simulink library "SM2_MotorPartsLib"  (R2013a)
settings: Solver=ode45  StartTime=0.0  StopTime=10.0  RelTol=1e-3
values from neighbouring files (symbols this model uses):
  m = v*BEAM.rho    [FlexBeamModelConstruct2.m]    (also in FlexBeamModelConstruct3.m = BEAM.rho*v; FlexBeam_1D_Construct.m = REF.m/REF.l*a.*(linspace(1-OPT.MassBiais+1e-6,1+OPT.MassBiai; FlexBeam_3D_Construct.m = REF.m/REF.l*a.*(linspace(1-OPT.MassBiais+1e-6,1+OPT.MassBiai; FreeFlexBeam_3D_Construct.m = REF.m/REF.l*a.*tmp2)
  N = D(1)+(H4^2+H3^2)/H2^2-(E(1)*H4+F(1)*H3)/H2    [MGD.m]    (also in MGD2.m)
  s = -sign(imag(KGZ_fr_tmp))    [LinprogReguliOptimFunc_1.m]    (also in LinprogReguliOptimFunc_2.m; LinprogReguliOptimFunc_1 - Copie.m)
  X = cos(phi(i))*x+sin(phi(i))*y    [MGI.m]
  Y = fft(y(:,i),NFFT)/L    [fft_bis.m]    (also in MGI.m = -sin(phi(i))*x+cos(phi(i))*y)
  Z = z    [MGI.m]
undefined symbols (not defined in the file or in its folder): AxisID, deg, kg, rad, SimParam
libraries: sm_lib x46, nesl_utility x13

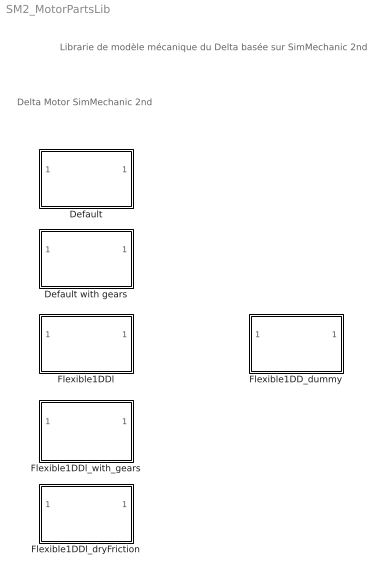
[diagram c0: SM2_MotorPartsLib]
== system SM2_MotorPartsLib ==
  note: Delta Motor SimMechanic 2nd
  note: Librarie de modèle mécanique du Delta basée sur SimMechanic 2nd
  Default : Subsystem  InitFcn=SimParam.Motor=RigidMotor_paramInitFnc(RawParam,IC);  VariantControl=motorVarDefault
  Default with gears : Subsystem  InitFcn=SimParam.Motor=RigidMotor_paramInitFnc(RawParam,IC);  VariantControl=motorVarGear
  Flexible1DD_dummy : Subsystem  InitFcn=SimParam.Motor=flexMotor_paramInitFnc(RawParam,IC);  VariantControl=motorVarFlex1
  Flexible1DDl : Subsystem  InitFcn=SimParam.Motor=flexMotor_paramInitFnc(RawParam,IC);  VariantControl=motorVarFlex1
  Flexible1DDl_dryFriction : Subsystem  InitFcn=SimParam.Motor=flexMotor_paramInitFnc(RawParam,IC);  VariantControl=motorVarFlex1
  Flexible1DDl_with_gears : Subsystem  InitFcn=SimParam.Motor=flexMotor_paramInitFnc(RawParam,IC);  VariantControl=motorVarFlex1

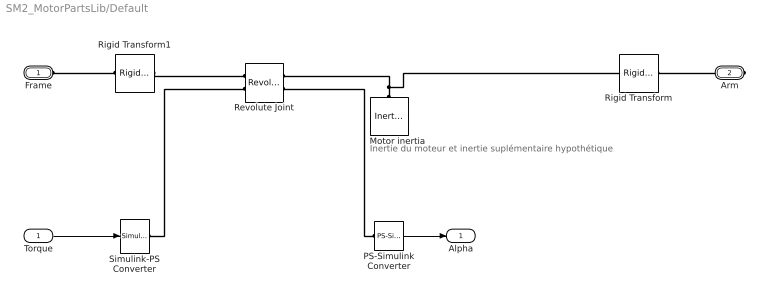
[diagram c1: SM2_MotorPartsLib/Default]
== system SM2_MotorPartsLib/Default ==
  note: Inertie du moteur et inertie suplémentaire hypothétique
  Torque : Inport
  Motor inertia : sm_lib/Body Elements/Inertia  InertiaType=Custom  Mass=1  MassUnits=kg  CenterOfMass=[0 0 0]  CenterOfMassUnits=m  MomentsOfInertia=(SimParam.Motor.I+SimParam.Motor.ISup).*[1 1 1]  MomentsOfInertiaUnits=kg*m^2  ProductsOfInertia=[0 0 0]  ProductsOfInertiaUnits=kg*m^2  BlockFunction=simmechanics.library.body_elements.inertia
  PS-Simulink Converter : nesl_utility/PS-Simulink Converter  PhysicalDomain=network_engine_domain  SubClassName=ps_output  LeftPortType=input  RightPortType=output  PseudoPeriodic=off  Frequencies=[]  Unit=1  AffineConversion=off
  Revolute Joint : sm_lib/Joints/Revolute Joint  SenseConstraintForceX=off  SenseConstraintForceY=off  SenseConstraintForceZ=off  SenseConstraintTorqueX=off  SenseConstraintTorqueY=off  SenseConstraintTorqueZ=off  ConstraintWrenchDir=FollowerOnBase  ConstraintWrenchFrame=BaseFrame  EquilibriumPosition=SimParam.Motor.Alpha(AxisID)  EquilibriumPositionUnits=rad  SpringStiffness=SimParam.Motor.kSup  SpringStiffnessUnits=N*m/rad  DampingCoefficient=SimParam.Motor.c  DampingCoefficientUnits=N*m/(rad/s)  ActuationMode=TorqueForceActuation  SensePosition=on  SenseVelocity=off  SenseAcceleration=off  SenseTorqueForce=off  PositionTargetValue=SimParam.Motor.Alpha(AxisID)  PositionTargetValueUnits=rad  PositionTargetSpecify=on  PositionTargetPriority=High  VelocityTargetValue=0  VelocityTargetValueUnits=rad/s  VelocityTargetSpecify=on  VelocityTargetPriority=High  BlockFunction=simmechanics.library.joints.revolute_joint
  Rigid Transform : sm_lib/Frames and  Transforms/Rigid  Transform  TranslationMethod=None  TranslationLengthUnit=m  TranslationStandardAxis=+Z  TranslationStandardOffset=0  TranslationCartesianOffset=[0 0 0]  TranslationROffset=0.2  TranslationROffsetUnits=m  TranslationZOffset=0  TranslationZOffsetUnits=m  TranslationThetaOffset=0  TranslationThetaOffsetUnits=deg  RotationMethod=AlignedAxes  RotationAngleUnits=rad  RotationStandardAxis=+Y  RotationAngle=0.2  RotationArbitraryAxis=[0 0 1]  FollAlignAxisA=+Y  BaseAlignAxisA=+Z  FollAlignAxisB=+X  BaseAlignAxisB=+X  BlockFunction=simmechanics.library.frames_transforms.rigid_transform
  Rigid Transform1 : sm_lib/Frames and  Transforms/Rigid  Transform  TranslationMethod=None  TranslationLengthUnit=m  TranslationStandardAxis=+Z  TranslationStandardOffset=0  TranslationCartesianOffset=[0 0 0]  TranslationROffset=0.2  TranslationROffsetUnits=m  TranslationZOffset=0  TranslationZOffsetUnits=m  TranslationThetaOffset=0  TranslationThetaOffsetUnits=deg  RotationMethod=AlignedAxes  RotationAngleUnits=rad  RotationStandardAxis=+Y  RotationAngle=0.2  RotationArbitraryAxis=[0 0 1]  FollAlignAxisA=+Z  BaseAlignAxisA=+Y  FollAlignAxisB=+X  BaseAlignAxisB=+X  BlockFunction=simmechanics.library.frames_transforms.rigid_transform
  Simulink-PS Converter : nesl_utility/Simulink-PS Converter  PhysicalDomain=network_engine_domain  SubClassName=ps_input  LeftPortType=input  RightPortType=output  PseudoPeriodic=off  Frequencies=[]  NoiseDistribution=none  NoiseParameters=[]  Unit=1  AffineConversion=off  InputFiltering=off  SimscapeFilterOrder=1  InputFilterTimeConstant=0.001  UdotUserProvided=1
  Frame : PMIOPort  Port=1  Side=Left
  Arm : PMIOPort  Port=2  Side=Right
  Alpha : Outport
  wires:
  PS-Simulink Converter/1 -> Alpha/1
  Torque/1 -> Simulink-PS Converter/1
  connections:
  Simulink-PS Converter/RConn1 -- Revolute Joint/LConn2
  Rigid Transform1/RConn1 -- Revolute Joint/LConn1
  Motor inertia/RConn1 -- Revolute Joint/RConn1 -- Rigid Transform/LConn1
  PS-Simulink Converter/LConn1 -- Revolute Joint/RConn2
  Rigid Transform1/LConn1 -- Frame/RConn1
  Arm/RConn1 -- Rigid Transform/RConn1

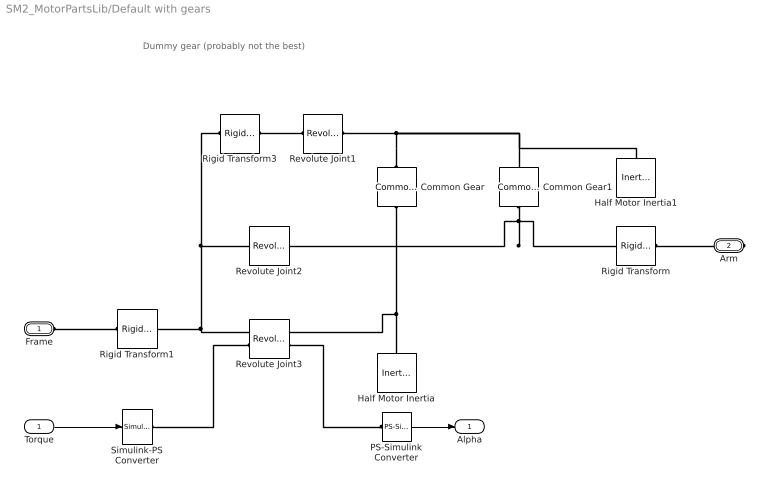
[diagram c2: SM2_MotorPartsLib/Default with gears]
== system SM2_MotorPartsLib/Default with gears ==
  note: Dummy gear (probably not the best)
  Torque : Inport
  Common Gear : sm_lib/Gears, Couplings and Drives/Gears/Common Gear  GearType=External  SpecificationType=CenterDistanceRatio  CenterDistance=0.01  CenterDistanceUnits=m  GearRatio=1  BaseGearRadius=10  BaseGearRadiusUnits=cm  FollGearRadius=10  FollGearRadiusUnits=cm  AssemblyGearRotation=Free  BlockFunction=simmechanics.library.gears_couplings_drives.gears.common_gear
  Common Gear1 : sm_lib/Gears, Couplings and Drives/Gears/Common Gear  GearType=External  SpecificationType=CenterDistanceRatio  CenterDistance=0.01  CenterDistanceUnits=m  GearRatio=SimParam.Motor.i  BaseGearRadius=10  BaseGearRadiusUnits=cm  FollGearRadius=10  FollGearRadiusUnits=cm  AssemblyGearRotation=Free  BlockFunction=simmechanics.library.gears_couplings_drives.gears.common_gear
  Half Motor Inertia : sm_lib/Body Elements/Inertia  InertiaType=Custom  Mass=1  MassUnits=kg  CenterOfMass=[0 0 0]  CenterOfMassUnits=m  MomentsOfInertia=0.5.*SimParam.Motor.I.*[1 1 1]  MomentsOfInertiaUnits=kg*m^2  ProductsOfInertia=[0 0 0]  ProductsOfInertiaUnits=kg*m^2  BlockFunction=simmechanics.library.body_elements.inertia
  Half Motor Inertia1 : sm_lib/Body Elements/Inertia  InertiaType=Custom  Mass=1  MassUnits=kg  CenterOfMass=[0 0 0]  CenterOfMassUnits=m  MomentsOfInertia=0.5.*SimParam.Motor.I.*[1 1 1]  MomentsOfInertiaUnits=kg*m^2  ProductsOfInertia=[0 0 0]  ProductsOfInertiaUnits=kg*m^2  BlockFunction=simmechanics.library.body_elements.inertia
  PS-Simulink Converter : nesl_utility/PS-Simulink Converter  PhysicalDomain=network_engine_domain  SubClassName=ps_output  LeftPortType=input  RightPortType=output  PseudoPeriodic=off  Frequencies=[]  Unit=1  AffineConversion=off
  Revolute Joint1 : sm_lib/Joints/Revolute Joint  SenseConstraintForceX=off  SenseConstraintForceY=off  SenseConstraintForceZ=off  SenseConstraintTorqueX=off  SenseConstraintTorqueY=off  SenseConstraintTorqueZ=off  ConstraintWrenchDir=FollowerOnBase  ConstraintWrenchFrame=BaseFrame  EquilibriumPosition=0  EquilibriumPositionUnits=rad  SpringStiffness=0  SpringStiffnessUnits=N*m/rad  DampingCoefficient=0  DampingCoefficientUnits=N*m/(rad/s)  ActuationMode=NoActuation  SensePosition=off  SenseVelocity=off  SenseAcceleration=off  SenseTorqueForce=off  PositionTargetValue=SimParam.Motor.Alpha(AxisID)  PositionTargetValueUnits=rad  PositionTargetSpecify=on  PositionTargetPriority=High  VelocityTargetValue=0  VelocityTargetValueUnits=deg/s  VelocityTargetSpecify=off  VelocityTargetPriority=High  BlockFunction=simmechanics.library.joints.revolute_joint
  Revolute Joint2 : sm_lib/Joints/Revolute Joint  SenseConstraintForceX=off  SenseConstraintForceY=off  SenseConstraintForceZ=off  SenseConstraintTorqueX=off  SenseConstraintTorqueY=off  SenseConstraintTorqueZ=off  ConstraintWrenchDir=FollowerOnBase  ConstraintWrenchFrame=BaseFrame  EquilibriumPosition=0  EquilibriumPositionUnits=rad  SpringStiffness=0  SpringStiffnessUnits=N*m/rad  DampingCoefficient=0  DampingCoefficientUnits=N*m/(rad/s)  ActuationMode=NoActuation  SensePosition=off  SenseVelocity=off  SenseAcceleration=off  SenseTorqueForce=off  PositionTargetValue=SimParam.Motor.Alpha(AxisID)  PositionTargetValueUnits=rad  PositionTargetSpecify=on  PositionTargetPriority=High  VelocityTargetValue=0  VelocityTargetValueUnits=deg/s  VelocityTargetSpecify=off  VelocityTargetPriority=High  BlockFunction=simmechanics.library.joints.revolute_joint
  Revolute Joint3 : sm_lib/Joints/Revolute Joint  SenseConstraintForceX=off  SenseConstraintForceY=off  SenseConstraintForceZ=off  SenseConstraintTorqueX=off  SenseConstraintTorqueY=off  SenseConstraintTorqueZ=off  ConstraintWrenchDir=FollowerOnBase  ConstraintWrenchFrame=BaseFrame  EquilibriumPosition=SimParam.IC.Alpha(AxisID)  EquilibriumPositionUnits=rad  SpringStiffness=SimParam.Motor.kSup  SpringStiffnessUnits=N*m/rad  DampingCoefficient=SimParam.Motor.c  DampingCoefficientUnits=N*m/(rad/s)  ActuationMode=TorqueForceActuation  SensePosition=on  SenseVelocity=off  SenseAcceleration=off  SenseTorqueForce=off  PositionTargetValue=SimParam.Motor.Alpha(AxisID)  PositionTargetValueUnits=rad  PositionTargetSpecify=on  PositionTargetPriority=High  VelocityTargetValue=0  VelocityTargetValueUnits=deg/s  VelocityTargetSpecify=off  VelocityTargetPriority=High  BlockFunction=simmechanics.library.joints.revolute_joint
  Rigid Transform : sm_lib/Frames and  Transforms/Rigid  Transform  TranslationMethod=None  TranslationLengthUnit=m  TranslationStandardAxis=+Z  TranslationStandardOffset=0  TranslationCartesianOffset=[0 0 0]  TranslationROffset=0.2  TranslationROffsetUnits=m  TranslationZOffset=0  TranslationZOffsetUnits=m  TranslationThetaOffset=0  TranslationThetaOffsetUnits=deg  RotationMethod=AlignedAxes  RotationAngleUnits=rad  RotationStandardAxis=+Y  RotationAngle=0.2  RotationArbitraryAxis=[0 0 1]  FollAlignAxisA=+Y  BaseAlignAxisA=+Z  FollAlignAxisB=+X  BaseAlignAxisB=+X  BlockFunction=simmechanics.library.frames_transforms.rigid_transform
  Rigid Transform1 : sm_lib/Frames and  Transforms/Rigid  Transform  TranslationMethod=None  TranslationLengthUnit=m  TranslationStandardAxis=+Z  TranslationStandardOffset=0  TranslationCartesianOffset=[0 0 0]  TranslationROffset=0.2  TranslationROffsetUnits=m  TranslationZOffset=0  TranslationZOffsetUnits=m  TranslationThetaOffset=0  TranslationThetaOffsetUnits=deg  RotationMethod=AlignedAxes  RotationAngleUnits=rad  RotationStandardAxis=+Y  RotationAngle=0.2  RotationArbitraryAxis=[0 0 1]  FollAlignAxisA=+Z  BaseAlignAxisA=+Y  FollAlignAxisB=+X  BaseAlignAxisB=+X  BlockFunction=simmechanics.library.frames_transforms.rigid_transform
  Rigid Transform3 : sm_lib/Frames and  Transforms/Rigid  Transform  TranslationMethod=Cartesian  TranslationLengthUnit=m  TranslationStandardAxis=+Z  TranslationStandardOffset=0  TranslationCartesianOffset=[0 .01 0]  TranslationROffset=0.2  TranslationROffsetUnits=m  TranslationZOffset=0  TranslationZOffsetUnits=m  TranslationThetaOffset=0  TranslationThetaOffsetUnits=deg  RotationMethod=None  RotationAngleUnits=rad  RotationStandardAxis=+Z  RotationAngle=SimParam.IC.Alpha(AxisID)  RotationArbitraryAxis=[0 0 1]  FollAlignAxisA=+Z  BaseAlignAxisA=+Y  FollAlignAxisB=+X  BaseAlignAxisB=+X  BlockFunction=simmechanics.library.frames_transforms.rigid_transform
  Simulink-PS Converter : nesl_utility/Simulink-PS Converter  PhysicalDomain=network_engine_domain  SubClassName=ps_input  LeftPortType=input  RightPortType=output  PseudoPeriodic=off  Frequencies=[]  NoiseDistribution=none  NoiseParameters=[]  Unit=1  AffineConversion=off  InputFiltering=off  SimscapeFilterOrder=1  InputFilterTimeConstant=0.001  UdotUserProvided=1
  Frame : PMIOPort  Port=1  Side=Left
  Arm : PMIOPort  Port=2  Side=Right
  Alpha : Outport
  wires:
  PS-Simulink Converter/1 -> Alpha/1
  Torque/1 -> Simulink-PS Converter/1
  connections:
  Revolute Joint3/LConn2 -- Simulink-PS Converter/RConn1
  Rigid Transform3/LConn1 -- Revolute Joint3/LConn1 -- Rigid Transform1/RConn1 -- Revolute Joint2/LConn1
  Common Gear/LConn1 -- Revolute Joint3/RConn1 -- Half Motor Inertia/RConn1
  Revolute Joint3/RConn2 -- PS-Simulink Converter/LConn1
  Rigid Transform1/LConn1 -- Frame/RConn1
  Common Gear/RConn1 -- Half Motor Inertia1/RConn1 -- Common Gear1/LConn1 -- Revolute Joint1/RConn1
  Revolute Joint1/LConn1 -- Rigid Transform3/RConn1
  Common Gear1/RConn1 -- Revolute Joint2/RConn1 -- Rigid Transform/LConn1
  Arm/RConn1 -- Rigid Transform/RConn1

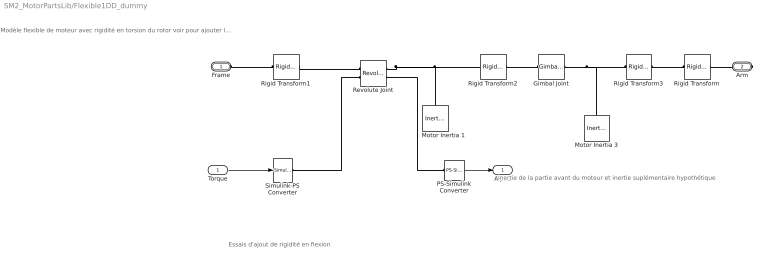
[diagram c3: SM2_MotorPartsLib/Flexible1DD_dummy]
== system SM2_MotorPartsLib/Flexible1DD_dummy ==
  note: Essais d'ajout de rigidité en flexion
  note: Modèle flexible de moteur avec rigidité en torsion du rotor voir pour ajouter le frottement sec éventuellement
  note: Inertie de la partie avant du moteur et inertie suplémentaire hypothétique
  Torque : Inport
  Gimbal Joint : sm_lib/Joints/Gimbal Joint  SenseConstraintForceX=off  SenseConstraintForceY=off  SenseConstraintForceZ=off  SenseConstraintTorqueX=off  SenseConstraintTorqueY=off  SenseConstraintTorqueZ=off  ConstraintWrenchDir=FollowerOnBase  ConstraintWrenchFrame=BaseFrame  RxEquilibriumPosition=0  RxEquilibriumPositionUnits=rad  RxSpringStiffness=SimParam.Motor.k*SimParam.Misc.DummyVal0  RxSpringStiffnessUnits=N*m/rad  RxDampingCoefficient=SimParam.Motor.c2*SimParam.Misc.DummyVal1  RxDampingCoefficientUnits=N*m/(rad/s)  RxActuationMode=NoActuation  RxSensePosition=off  RxSenseVelocity=off  RxSenseAcceleration=off  RxSenseTorqueForce=off  RxPositionTargetValue=0  RxPositionTargetValueUnits=deg  RxPositionTargetSpecify=on  RxPositionTargetPriority=High  RxVelocityTargetValue=0  RxVelocityTargetValueUnits=deg/s  RxVelocityTargetSpecify=on  RxVelocityTargetPriority=High  RyEquilibriumPosition=0  RyEquilibriumPositionUnits=rad  RySpringStiffness=SimParam.Motor.k*SimParam.Misc.DummyVal0  RySpringStiffnessUnits=N*m/rad  RyDampingCoefficient=SimParam.Motor.c2*SimParam.Misc.DummyVal1  RyDampingCoefficientUnits=N*m/(rad/s)  RyActuationMode=NoActuation  RySensePosition=off  RySenseVelocity=off  RySenseAcceleration=off  RySenseTorqueForce=off  RyPositionTargetValue=0  RyPositionTargetValueUnits=deg  RyPositionTargetSpecify=on  RyPositionTargetPriority=High  RyVelocityTargetValue=0  RyVelocityTargetValueUnits=deg/s  RyVelocityTargetSpecify=on  RyVelocityTargetPriority=High  RzEquilibriumPosition=0  RzEquilibriumPositionUnits=rad  RzSpringStiffness=SimParam.Motor.k  RzSpringStiffnessUnits=N*m/rad  RzDampingCoefficient=SimParam.Motor.c2  RzDampingCoefficientUnits=N*m/(rad/s)  RzActuationMode=NoActuation  RzSensePosition=off  RzSenseVelocity=off  RzSenseAcceleration=off  RzSenseTorqueForce=off  RzPositionTargetValue=0  RzPositionTargetValueUnits=deg  RzPositionTargetSpecify=on  RzPositionTargetPriority=High  RzVelocityTargetValue=0  RzVelocityTargetValueUnits=deg/s  RzVelocityTargetSpecify=on  RzVelocityTargetPriority=High  BlockFunction=simmechanics.library.joints.gimbal_joint
  Motor Inertia 1 : sm_lib/Body Elements/Inertia  InertiaType=Custom  Mass=1  MassUnits=kg  CenterOfMass=[0 0 0]  CenterOfMassUnits=m  MomentsOfInertia=SimParam.Motor.I(1).*[1 1 1]  MomentsOfInertiaUnits=kg*m^2  ProductsOfInertia=[0 0 0]  ProductsOfInertiaUnits=kg*m^2  BlockFunction=simmechanics.library.body_elements.inertia
  Motor Inertia 3 : sm_lib/Body Elements/Inertia  InertiaType=Custom  Mass=0.1  MassUnits=kg  CenterOfMass=[0 0 0]  CenterOfMassUnits=m  MomentsOfInertia=(SimParam.Motor.I(2)+SimParam.Motor.ISup).*[0.1 0.1 1]  MomentsOfInertiaUnits=kg*m^2  ProductsOfInertia=[0 0 0]  ProductsOfInertiaUnits=kg*m^2  BlockFunction=simmechanics.library.body_elements.inertia
  PS-Simulink Converter : nesl_utility/PS-Simulink Converter  PhysicalDomain=network_engine_domain  SubClassName=ps_output  LeftPortType=input  RightPortType=output  PseudoPeriodic=off  Frequencies=[]  Unit=1  AffineConversion=off
  Revolute Joint : sm_lib/Joints/Revolute Joint  SenseConstraintForceX=off  SenseConstraintForceY=off  SenseConstraintForceZ=off  SenseConstraintTorqueX=off  SenseConstraintTorqueY=off  SenseConstraintTorqueZ=off  ConstraintWrenchDir=FollowerOnBase  ConstraintWrenchFrame=BaseFrame  EquilibriumPosition=SimParam.Motor.Alpha(AxisID)  EquilibriumPositionUnits=rad  SpringStiffness=SimParam.Motor.kSup  SpringStiffnessUnits=N*m/rad  DampingCoefficient=SimParam.Motor.c  DampingCoefficientUnits=N*m/(rad/s)  ActuationMode=TorqueForceActuation  SensePosition=on  SenseVelocity=off  SenseAcceleration=off  SenseTorqueForce=off  PositionTargetValue=SimParam.Motor.Alpha(AxisID)  PositionTargetValueUnits=rad  PositionTargetSpecify=on  PositionTargetPriority=Low  VelocityTargetValue=0  VelocityTargetValueUnits=rad/s  VelocityTargetSpecify=on  VelocityTargetPriority=High  BlockFunction=simmechanics.library.joints.revolute_joint
  Rigid Transform : sm_lib/Frames and  Transforms/Rigid  Transform  TranslationMethod=None  TranslationLengthUnit=m  TranslationStandardAxis=+Z  TranslationStandardOffset=0  TranslationCartesianOffset=[0 0 0]  TranslationROffset=0.2  TranslationROffsetUnits=m  TranslationZOffset=0  TranslationZOffsetUnits=m  TranslationThetaOffset=0  TranslationThetaOffsetUnits=deg  RotationMethod=AlignedAxes  RotationAngleUnits=rad  RotationStandardAxis=+Y  RotationAngle=0.2  RotationArbitraryAxis=[0 0 1]  FollAlignAxisA=+Y  BaseAlignAxisA=+Z  FollAlignAxisB=+X  BaseAlignAxisB=+X  BlockFunction=simmechanics.library.frames_transforms.rigid_transform
  Rigid Transform1 : sm_lib/Frames and  Transforms/Rigid  Transform  TranslationMethod=None  TranslationLengthUnit=m  TranslationStandardAxis=+Z  TranslationStandardOffset=0  TranslationCartesianOffset=[0 0 0]  TranslationROffset=0.2  TranslationROffsetUnits=m  TranslationZOffset=0  TranslationZOffsetUnits=m  TranslationThetaOffset=0  TranslationThetaOffsetUnits=deg  RotationMethod=AlignedAxes  RotationAngleUnits=rad  RotationStandardAxis=+Y  RotationAngle=0.2  RotationArbitraryAxis=[0 0 1]  FollAlignAxisA=+Z  BaseAlignAxisA=+Y  FollAlignAxisB=+X  BaseAlignAxisB=+X  BlockFunction=simmechanics.library.frames_transforms.rigid_transform
  Rigid Transform2 : sm_lib/Frames and  Transforms/Rigid  Transform  TranslationMethod=Cartesian  TranslationLengthUnit=m  TranslationStandardAxis=+Z  TranslationStandardOffset=0  TranslationCartesianOffset=[0 0 -SimParam.Misc.DummyVal2]  TranslationROffset=0.2  TranslationROffsetUnits=m  TranslationZOffset=0  TranslationZOffsetUnits=m  TranslationThetaOffset=0  TranslationThetaOffsetUnits=deg  RotationMethod=None  RotationAngleUnits=rad  RotationStandardAxis=+Y  RotationAngle=0.2  RotationArbitraryAxis=[0 0 1]  FollAlignAxisA=+Z  BaseAlignAxisA=+Y  FollAlignAxisB=+X  BaseAlignAxisB=+X  BlockFunction=simmechanics.library.frames_transforms.rigid_transform
  Rigid Transform3 : sm_lib/Frames and  Transforms/Rigid  Transform  TranslationMethod=Cartesian  TranslationLengthUnit=m  TranslationStandardAxis=+Z  TranslationStandardOffset=0  TranslationCartesianOffset=[0 0 SimParam.Misc.DummyVal2]  TranslationROffset=0.2  TranslationROffsetUnits=m  TranslationZOffset=0  TranslationZOffsetUnits=m  TranslationThetaOffset=0  TranslationThetaOffsetUnits=deg  RotationMethod=None  RotationAngleUnits=rad  RotationStandardAxis=+Y  RotationAngle=0.2  RotationArbitraryAxis=[0 0 1]  FollAlignAxisA=+Z  BaseAlignAxisA=+Y  FollAlignAxisB=+X  BaseAlignAxisB=+X  BlockFunction=simmechanics.library.frames_transforms.rigid_transform
  Simulink-PS Converter : nesl_utility/Simulink-PS Converter  PhysicalDomain=network_engine_domain  SubClassName=ps_input  LeftPortType=input  RightPortType=output  PseudoPeriodic=off  Frequencies=[]  NoiseDistribution=none  NoiseParameters=[]  Unit=1  AffineConversion=off  InputFiltering=off  SimscapeFilterOrder=1  InputFilterTimeConstant=0.001  UdotUserProvided=1
  Frame : PMIOPort  Port=1  Side=Left
  Arm : PMIOPort  Port=2  Side=Right
  Alpha : Outport
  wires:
  PS-Simulink Converter/1 -> Alpha/1
  Torque/1 -> Simulink-PS Converter/1
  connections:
  Rigid Transform/RConn1 -- Arm/RConn1
  Revolute Joint/RConn1 -- Rigid Transform2/LConn1 -- Motor Inertia 1/RConn1
  Simulink-PS Converter/RConn1 -- Revolute Joint/LConn2
  PS-Simulink Converter/LConn1 -- Revolute Joint/RConn2
  Rigid Transform1/RConn1 -- Revolute Joint/LConn1
  Frame/RConn1 -- Rigid Transform1/LConn1
  Gimbal Joint/LConn1 -- Rigid Transform2/RConn1
  Gimbal Joint/RConn1 -- Motor Inertia 3/RConn1 -- Rigid Transform3/LConn1
  Rigid Transform/LConn1 -- Rigid Transform3/RConn1

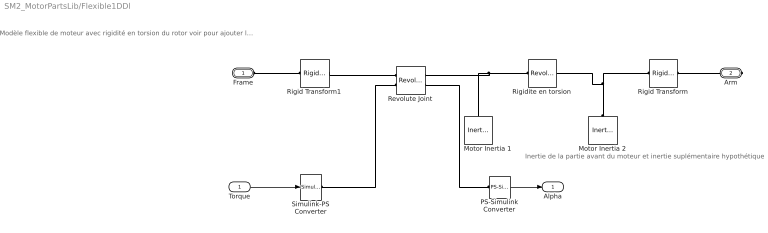
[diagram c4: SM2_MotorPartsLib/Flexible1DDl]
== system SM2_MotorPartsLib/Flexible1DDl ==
  note: Modèle flexible de moteur avec rigidité en torsion du rotor voir pour ajouter le frottement sec éventuellement
  note: Inertie de la partie avant du moteur et inertie suplémentaire hypothétique
  Torque : Inport
  Motor Inertia 1 : sm_lib/Body Elements/Inertia  InertiaType=Custom  Mass=1  MassUnits=kg  CenterOfMass=[0 0 0]  CenterOfMassUnits=m  MomentsOfInertia=SimParam.Motor.I(1).*[1 1 1]  MomentsOfInertiaUnits=kg*m^2  ProductsOfInertia=[0 0 0]  ProductsOfInertiaUnits=kg*m^2  BlockFunction=simmechanics.library.body_elements.inertia
  Motor Inertia 2 : sm_lib/Body Elements/Inertia  InertiaType=Custom  Mass=1  MassUnits=kg  CenterOfMass=[0 0 0]  CenterOfMassUnits=m  MomentsOfInertia=(SimParam.Motor.I(2)+SimParam.Motor.ISup).*[1 1 1]  MomentsOfInertiaUnits=kg*m^2  ProductsOfInertia=[0 0 0]  ProductsOfInertiaUnits=kg*m^2  BlockFunction=simmechanics.library.body_elements.inertia
  PS-Simulink Converter : nesl_utility/PS-Simulink Converter  PhysicalDomain=network_engine_domain  SubClassName=ps_output  LeftPortType=input  RightPortType=output  PseudoPeriodic=off  Frequencies=[]  Unit=1  AffineConversion=off
  Revolute Joint : sm_lib/Joints/Revolute Joint  SenseConstraintForceX=off  SenseConstraintForceY=off  SenseConstraintForceZ=off  SenseConstraintTorqueX=off  SenseConstraintTorqueY=off  SenseConstraintTorqueZ=off  ConstraintWrenchDir=FollowerOnBase  ConstraintWrenchFrame=BaseFrame  EquilibriumPosition=SimParam.Motor.Alpha(AxisID)  EquilibriumPositionUnits=rad  SpringStiffness=SimParam.Motor.kSup  SpringStiffnessUnits=N*m/rad  DampingCoefficient=SimParam.Motor.c  DampingCoefficientUnits=N*m/(rad/s)  ActuationMode=TorqueForceActuation  SensePosition=on  SenseVelocity=off  SenseAcceleration=off  SenseTorqueForce=off  PositionTargetValue=SimParam.Motor.Alpha(AxisID)  PositionTargetValueUnits=rad  PositionTargetSpecify=on  PositionTargetPriority=Low  VelocityTargetValue=0  VelocityTargetValueUnits=rad/s  VelocityTargetSpecify=on  VelocityTargetPriority=High  BlockFunction=simmechanics.library.joints.revolute_joint
  Rigid Transform : sm_lib/Frames and  Transforms/Rigid  Transform  TranslationMethod=None  TranslationLengthUnit=m  TranslationStandardAxis=+Z  TranslationStandardOffset=0  TranslationCartesianOffset=[0 0 0]  TranslationROffset=0.2  TranslationROffsetUnits=m  TranslationZOffset=0  TranslationZOffsetUnits=m  TranslationThetaOffset=0  TranslationThetaOffsetUnits=deg  RotationMethod=AlignedAxes  RotationAngleUnits=rad  RotationStandardAxis=+Y  RotationAngle=0.2  RotationArbitraryAxis=[0 0 1]  FollAlignAxisA=+Y  BaseAlignAxisA=+Z  FollAlignAxisB=+X  BaseAlignAxisB=+X  BlockFunction=simmechanics.library.frames_transforms.rigid_transform
  Rigid Transform1 : sm_lib/Frames and  Transforms/Rigid  Transform  TranslationMethod=None  TranslationLengthUnit=m  TranslationStandardAxis=+Z  TranslationStandardOffset=0  TranslationCartesianOffset=[0 0 0]  TranslationROffset=0.2  TranslationROffsetUnits=m  TranslationZOffset=0  TranslationZOffsetUnits=m  TranslationThetaOffset=0  TranslationThetaOffsetUnits=deg  RotationMethod=AlignedAxes  RotationAngleUnits=rad  RotationStandardAxis=+Y  RotationAngle=0.2  RotationArbitraryAxis=[0 0 1]  FollAlignAxisA=+Z  BaseAlignAxisA=+Y  FollAlignAxisB=+X  BaseAlignAxisB=+X  BlockFunction=simmechanics.library.frames_transforms.rigid_transform
  Rigidite en torsion : sm_lib/Joints/Revolute Joint  SenseConstraintForceX=off  SenseConstraintForceY=off  SenseConstraintForceZ=off  SenseConstraintTorqueX=off  SenseConstraintTorqueY=off  SenseConstraintTorqueZ=off  ConstraintWrenchDir=FollowerOnBase  ConstraintWrenchFrame=BaseFrame  EquilibriumPosition=0  EquilibriumPositionUnits=rad  SpringStiffness=SimParam.Motor.k  SpringStiffnessUnits=N*m/rad  DampingCoefficient=SimParam.Motor.c2  DampingCoefficientUnits=N*m/(rad/s)  ActuationMode=NoActuation  SensePosition=off  SenseVelocity=off  SenseAcceleration=off  SenseTorqueForce=off  PositionTargetValue=0  PositionTargetValueUnits=rad  PositionTargetSpecify=on  PositionTargetPriority=High  VelocityTargetValue=0  VelocityTargetValueUnits=rad/s  VelocityTargetSpecify=on  VelocityTargetPriority=High  BlockFunction=simmechanics.library.joints.revolute_joint
  Simulink-PS Converter : nesl_utility/Simulink-PS Converter  PhysicalDomain=network_engine_domain  SubClassName=ps_input  LeftPortType=input  RightPortType=output  PseudoPeriodic=off  Frequencies=[]  NoiseDistribution=none  NoiseParameters=[]  Unit=1  AffineConversion=off  InputFiltering=off  SimscapeFilterOrder=1  InputFilterTimeConstant=0.001  UdotUserProvided=1
  Frame : PMIOPort  Port=1  Side=Left
  Arm : PMIOPort  Port=2  Side=Right
  Alpha : Outport
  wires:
  PS-Simulink Converter/1 -> Alpha/1
  Torque/1 -> Simulink-PS Converter/1
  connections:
  Rigid Transform/RConn1 -- Arm/RConn1
  Rigidite en torsion/LConn1 -- Revolute Joint/RConn1 -- Motor Inertia 1/RConn1
  Motor Inertia 2/RConn1 -- Rigid Transform/LConn1 -- Rigidite en torsion/RConn1
  Simulink-PS Converter/RConn1 -- Revolute Joint/LConn2
  PS-Simulink Converter/LConn1 -- Revolute Joint/RConn2
  Rigid Transform1/RConn1 -- Revolute Joint/LConn1
  Frame/RConn1 -- Rigid Transform1/LConn1

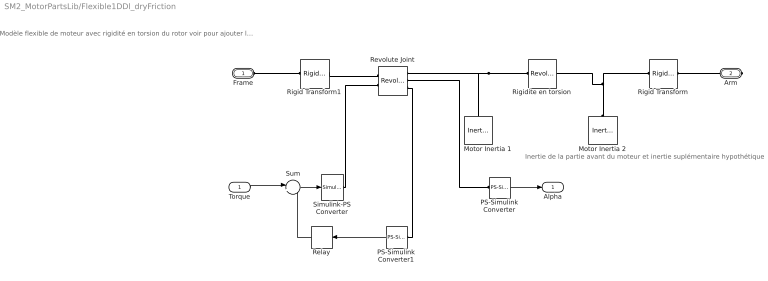
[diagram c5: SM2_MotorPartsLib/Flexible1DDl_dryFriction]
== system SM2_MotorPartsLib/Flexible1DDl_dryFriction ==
  note: Modèle flexible de moteur avec rigidité en torsion du rotor voir pour ajouter le frottement sec éventuellement
  note: Inertie de la partie avant du moteur et inertie suplémentaire hypothétique
  Torque : Inport
  Motor Inertia 1 : sm_lib/Body Elements/Inertia  InertiaType=Custom  Mass=1  MassUnits=kg  CenterOfMass=[0 0 0]  CenterOfMassUnits=m  MomentsOfInertia=SimParam.Motor.I(1).*[1 1 1]  MomentsOfInertiaUnits=kg*m^2  ProductsOfInertia=[0 0 0]  ProductsOfInertiaUnits=kg*m^2  BlockFunction=simmechanics.library.body_elements.inertia
  Motor Inertia 2 : sm_lib/Body Elements/Inertia  InertiaType=Custom  Mass=1  MassUnits=kg  CenterOfMass=[0 0 0]  CenterOfMassUnits=m  MomentsOfInertia=(SimParam.Motor.I(2)+SimParam.Motor.ISup).*[1 1 1]  MomentsOfInertiaUnits=kg*m^2  ProductsOfInertia=[0 0 0]  ProductsOfInertiaUnits=kg*m^2  BlockFunction=simmechanics.library.body_elements.inertia
  PS-Simulink Converter : nesl_utility/PS-Simulink Converter  PhysicalDomain=network_engine_domain  SubClassName=ps_output  LeftPortType=input  RightPortType=output  PseudoPeriodic=off  Frequencies=[]  Unit=1  AffineConversion=off
  PS-Simulink Converter1 : nesl_utility/PS-Simulink Converter  PhysicalDomain=network_engine_domain  SubClassName=ps_output  LeftPortType=input  RightPortType=output  PseudoPeriodic=off  Frequencies=[]  Unit=1  AffineConversion=off
  Relay : Relay  OnSwitchValue=1e-3  OffSwitchValue=-1e-3  OnOutputValue=SimParam.Motor.cd  OffOutputValue=-SimParam.Motor.cd
  Revolute Joint : sm_lib/Joints/Revolute Joint  SenseConstraintForceX=off  SenseConstraintForceY=off  SenseConstraintForceZ=off  SenseConstraintTorqueX=off  SenseConstraintTorqueY=off  SenseConstraintTorqueZ=off  ConstraintWrenchDir=FollowerOnBase  ConstraintWrenchFrame=BaseFrame  EquilibriumPosition=SimParam.Motor.Alpha(AxisID)  EquilibriumPositionUnits=rad  SpringStiffness=SimParam.Motor.kSup  SpringStiffnessUnits=N*m/rad  DampingCoefficient=SimParam.Motor.c  DampingCoefficientUnits=N*m/(rad/s)  ActuationMode=TorqueForceActuation  SensePosition=on  SenseVelocity=on  SenseAcceleration=off  SenseTorqueForce=off  PositionTargetValue=SimParam.Motor.Alpha(AxisID)  PositionTargetValueUnits=rad  PositionTargetSpecify=on  PositionTargetPriority=High  VelocityTargetValue=0  VelocityTargetValueUnits=rad/s  VelocityTargetSpecify=on  VelocityTargetPriority=High  BlockFunction=simmechanics.library.joints.revolute_joint
  Rigid Transform : sm_lib/Frames and  Transforms/Rigid  Transform  TranslationMethod=None  TranslationLengthUnit=m  TranslationStandardAxis=+Z  TranslationStandardOffset=0  TranslationCartesianOffset=[0 0 0]  TranslationROffset=0.2  TranslationROffsetUnits=m  TranslationZOffset=0  TranslationZOffsetUnits=m  TranslationThetaOffset=0  TranslationThetaOffsetUnits=deg  RotationMethod=AlignedAxes  RotationAngleUnits=rad  RotationStandardAxis=+Y  RotationAngle=0.2  RotationArbitraryAxis=[0 0 1]  FollAlignAxisA=+Y  BaseAlignAxisA=+Z  FollAlignAxisB=+X  BaseAlignAxisB=+X  BlockFunction=simmechanics.library.frames_transforms.rigid_transform
  Rigid Transform1 : sm_lib/Frames and  Transforms/Rigid  Transform  TranslationMethod=None  TranslationLengthUnit=m  TranslationStandardAxis=+Z  TranslationStandardOffset=0  TranslationCartesianOffset=[0 0 0]  TranslationROffset=0.2  TranslationROffsetUnits=m  TranslationZOffset=0  TranslationZOffsetUnits=m  TranslationThetaOffset=0  TranslationThetaOffsetUnits=deg  RotationMethod=AlignedAxes  RotationAngleUnits=rad  RotationStandardAxis=+Y  RotationAngle=0.2  RotationArbitraryAxis=[0 0 1]  FollAlignAxisA=+Z  BaseAlignAxisA=+Y  FollAlignAxisB=+X  BaseAlignAxisB=+X  BlockFunction=simmechanics.library.frames_transforms.rigid_transform
  Rigidite en torsion : sm_lib/Joints/Revolute Joint  SenseConstraintForceX=off  SenseConstraintForceY=off  SenseConstraintForceZ=off  SenseConstraintTorqueX=off  SenseConstraintTorqueY=off  SenseConstraintTorqueZ=off  ConstraintWrenchDir=FollowerOnBase  ConstraintWrenchFrame=BaseFrame  EquilibriumPosition=0  EquilibriumPositionUnits=rad  SpringStiffness=SimParam.Motor.k  SpringStiffnessUnits=N*m/rad  DampingCoefficient=SimParam.Motor.c2  DampingCoefficientUnits=N*m/(rad/s)  ActuationMode=NoActuation  SensePosition=off  SenseVelocity=off  SenseAcceleration=off  SenseTorqueForce=off  PositionTargetValue=0  PositionTargetValueUnits=rad  PositionTargetSpecify=on  PositionTargetPriority=High  VelocityTargetValue=0  VelocityTargetValueUnits=rad/s  VelocityTargetSpecify=on  VelocityTargetPriority=High  BlockFunction=simmechanics.library.joints.revolute_joint
  Simulink-PS Converter : nesl_utility/Simulink-PS Converter  PhysicalDomain=network_engine_domain  SubClassName=ps_input  LeftPortType=input  RightPortType=output  PseudoPeriodic=off  Frequencies=[]  NoiseDistribution=none  NoiseParameters=[]  Unit=1  AffineConversion=off  InputFiltering=off  SimscapeFilterOrder=1  InputFilterTimeConstant=0.001  UdotUserProvided=1
  Sum : Sum  Inputs=|+-
  Frame : PMIOPort  Port=1  Side=Left
  Arm : PMIOPort  Port=2  Side=Right
  Alpha : Outport
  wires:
  PS-Simulink Converter/1 -> Alpha/1
  Torque/1 -> Sum/1
  Sum/1 -> Simulink-PS Converter/1
  PS-Simulink Converter1/1 -> Relay/1
  Relay/1 -> Sum/2
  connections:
  Rigid Transform/RConn1 -- Arm/RConn1
  Rigidite en torsion/LConn1 -- Revolute Joint/RConn1 -- Motor Inertia 1/RConn1
  Motor Inertia 2/RConn1 -- Rigid Transform/LConn1 -- Rigidite en torsion/RConn1
  Simulink-PS Converter/RConn1 -- Revolute Joint/LConn2
  PS-Simulink Converter/LConn1 -- Revolute Joint/RConn2
  Rigid Transform1/RConn1 -- Revolute Joint/LConn1
  Frame/RConn1 -- Rigid Transform1/LConn1
  PS-Simulink Converter1/LConn1 -- Revolute Joint/RConn3

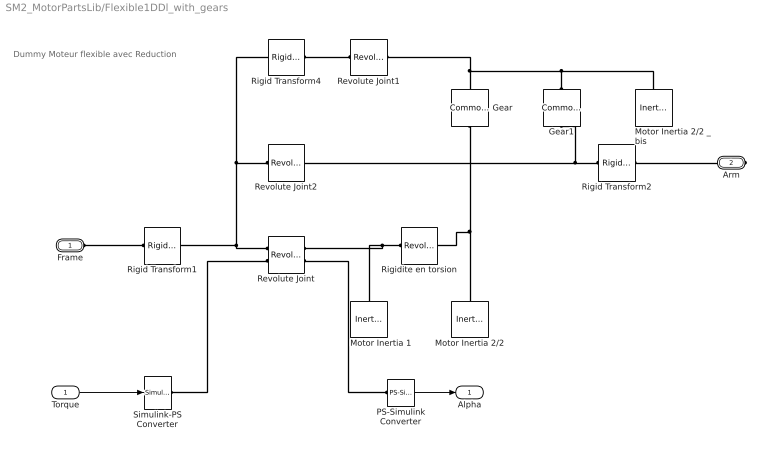
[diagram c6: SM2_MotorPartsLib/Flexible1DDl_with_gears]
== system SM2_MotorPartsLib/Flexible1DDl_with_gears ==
  note: Dummy Moteur flexible avec Reduction
  Torque : Inport
  Gear : sm_lib/Gears, Couplings and Drives/Gears/Common Gear  GearType=External  SpecificationType=CenterDistanceRatio  CenterDistance=0.01  CenterDistanceUnits=m  GearRatio=1  BaseGearRadius=10  BaseGearRadiusUnits=cm  FollGearRadius=10  FollGearRadiusUnits=cm  AssemblyGearRotation=Free  BlockFunction=simmechanics.library.gears_couplings_drives.gears.common_gear
  Gear1 : sm_lib/Gears, Couplings and Drives/Gears/Common Gear  GearType=External  SpecificationType=CenterDistanceRatio  CenterDistance=0.01  CenterDistanceUnits=m  GearRatio=SimParam.Motor.i  BaseGearRadius=10  BaseGearRadiusUnits=cm  FollGearRadius=10  FollGearRadiusUnits=cm  AssemblyGearRotation=Free  BlockFunction=simmechanics.library.gears_couplings_drives.gears.common_gear
  Motor Inertia 1 : sm_lib/Body Elements/Inertia  InertiaType=Custom  Mass=1  MassUnits=kg  CenterOfMass=[0 0 0]  CenterOfMassUnits=m  MomentsOfInertia=SimParam.Motor.I(1).*[1 1 1]  MomentsOfInertiaUnits=kg*m^2  ProductsOfInertia=[0 0 0]  ProductsOfInertiaUnits=kg*m^2  BlockFunction=simmechanics.library.body_elements.inertia
  Motor Inertia 2/2 : sm_lib/Body Elements/Inertia  InertiaType=Custom  Mass=1  MassUnits=kg  CenterOfMass=[0 0 0]  CenterOfMassUnits=m  MomentsOfInertia=0.5*(SimParam.Motor.I(2)+SimParam.Motor.ISup).*[1 1 1]  MomentsOfInertiaUnits=kg*m^2  ProductsOfInertia=[0 0 0]  ProductsOfInertiaUnits=kg*m^2  BlockFunction=simmechanics.library.body_elements.inertia
  Motor Inertia 2/2 _bis : sm_lib/Body Elements/Inertia  InertiaType=Custom  Mass=1  MassUnits=kg  CenterOfMass=[0 0 0]  CenterOfMassUnits=m  MomentsOfInertia=0.5*(SimParam.Motor.I(2)+SimParam.Motor.ISup).*[1 1 1]  MomentsOfInertiaUnits=kg*m^2  ProductsOfInertia=[0 0 0]  ProductsOfInertiaUnits=kg*m^2  BlockFunction=simmechanics.library.body_elements.inertia
  PS-Simulink Converter : nesl_utility/PS-Simulink Converter  PhysicalDomain=network_engine_domain  SubClassName=ps_output  LeftPortType=input  RightPortType=output  PseudoPeriodic=off  Frequencies=[]  Unit=1  AffineConversion=off
  Revolute Joint : sm_lib/Joints/Revolute Joint  SenseConstraintForceX=off  SenseConstraintForceY=off  SenseConstraintForceZ=off  SenseConstraintTorqueX=off  SenseConstraintTorqueY=off  SenseConstraintTorqueZ=off  ConstraintWrenchDir=FollowerOnBase  ConstraintWrenchFrame=BaseFrame  EquilibriumPosition=SimParam.Motor.Alpha(AxisID)  EquilibriumPositionUnits=rad  SpringStiffness=SimParam.Motor.kSup  SpringStiffnessUnits=N*m/rad  DampingCoefficient=SimParam.Motor.c  DampingCoefficientUnits=N*m/(rad/s)  ActuationMode=TorqueForceActuation  SensePosition=on  SenseVelocity=off  SenseAcceleration=off  SenseTorqueForce=off  PositionTargetValue=SimParam.Motor.Alpha(AxisID)  PositionTargetValueUnits=rad  PositionTargetSpecify=on  PositionTargetPriority=Low  VelocityTargetValue=0  VelocityTargetValueUnits=rad/s  VelocityTargetSpecify=on  VelocityTargetPriority=High  BlockFunction=simmechanics.library.joints.revolute_joint
  Revolute Joint1 : sm_lib/Joints/Revolute Joint  SenseConstraintForceX=off  SenseConstraintForceY=off  SenseConstraintForceZ=off  SenseConstraintTorqueX=off  SenseConstraintTorqueY=off  SenseConstraintTorqueZ=off  ConstraintWrenchDir=FollowerOnBase  ConstraintWrenchFrame=BaseFrame  EquilibriumPosition=0  EquilibriumPositionUnits=rad  SpringStiffness=0  SpringStiffnessUnits=N*m/rad  DampingCoefficient=0  DampingCoefficientUnits=N*m/(rad/s)  ActuationMode=NoActuation  SensePosition=off  SenseVelocity=off  SenseAcceleration=off  SenseTorqueForce=off  PositionTargetValue=SimParam.Motor.Alpha(AxisID)  PositionTargetValueUnits=rad  PositionTargetSpecify=on  PositionTargetPriority=High  VelocityTargetValue=0  VelocityTargetValueUnits=deg/s  VelocityTargetSpecify=off  VelocityTargetPriority=High  BlockFunction=simmechanics.library.joints.revolute_joint
  Revolute Joint2 : sm_lib/Joints/Revolute Joint  SenseConstraintForceX=off  SenseConstraintForceY=off  SenseConstraintForceZ=off  SenseConstraintTorqueX=off  SenseConstraintTorqueY=off  SenseConstraintTorqueZ=off  ConstraintWrenchDir=FollowerOnBase  ConstraintWrenchFrame=BaseFrame  EquilibriumPosition=0  EquilibriumPositionUnits=rad  SpringStiffness=0  SpringStiffnessUnits=N*m/rad  DampingCoefficient=0  DampingCoefficientUnits=N*m/(rad/s)  ActuationMode=NoActuation  SensePosition=off  SenseVelocity=off  SenseAcceleration=off  SenseTorqueForce=off  PositionTargetValue=SimParam.Motor.Alpha(AxisID)  PositionTargetValueUnits=rad  PositionTargetSpecify=on  PositionTargetPriority=High  VelocityTargetValue=0  VelocityTargetValueUnits=deg/s  VelocityTargetSpecify=off  VelocityTargetPriority=High  BlockFunction=simmechanics.library.joints.revolute_joint
  Rigid Transform1 : sm_lib/Frames and  Transforms/Rigid  Transform  TranslationMethod=None  TranslationLengthUnit=m  TranslationStandardAxis=+Z  TranslationStandardOffset=0  TranslationCartesianOffset=[0 0 0]  TranslationROffset=0.2  TranslationROffsetUnits=m  TranslationZOffset=0  TranslationZOffsetUnits=m  TranslationThetaOffset=0  TranslationThetaOffsetUnits=deg  RotationMethod=AlignedAxes  RotationAngleUnits=rad  RotationStandardAxis=+Y  RotationAngle=0.2  RotationArbitraryAxis=[0 0 1]  FollAlignAxisA=+Z  BaseAlignAxisA=+Y  FollAlignAxisB=+X  BaseAlignAxisB=+X  BlockFunction=simmechanics.library.frames_transforms.rigid_transform
  Rigid Transform2 : sm_lib/Frames and  Transforms/Rigid  Transform  TranslationMethod=None  TranslationLengthUnit=m  TranslationStandardAxis=+Z  TranslationStandardOffset=0  TranslationCartesianOffset=[0 0 0]  TranslationROffset=0.2  TranslationROffsetUnits=m  TranslationZOffset=0  TranslationZOffsetUnits=m  TranslationThetaOffset=0  TranslationThetaOffsetUnits=deg  RotationMethod=AlignedAxes  RotationAngleUnits=rad  RotationStandardAxis=+Y  RotationAngle=0.2  RotationArbitraryAxis=[0 0 1]  FollAlignAxisA=+Y  BaseAlignAxisA=+Z  FollAlignAxisB=+X  BaseAlignAxisB=+X  BlockFunction=simmechanics.library.frames_transforms.rigid_transform
  Rigid Transform4 : sm_lib/Frames and  Transforms/Rigid  Transform  TranslationMethod=Cartesian  TranslationLengthUnit=m  TranslationStandardAxis=+Z  TranslationStandardOffset=0  TranslationCartesianOffset=[0 .01 0]  TranslationROffset=0.2  TranslationROffsetUnits=m  TranslationZOffset=0  TranslationZOffsetUnits=m  TranslationThetaOffset=0  TranslationThetaOffsetUnits=deg  RotationMethod=None  RotationAngleUnits=rad  RotationStandardAxis=+Z  RotationAngle=SimParam.IC.Alpha(AxisID)  RotationArbitraryAxis=[0 0 1]  FollAlignAxisA=+Z  BaseAlignAxisA=+Y  FollAlignAxisB=+X  BaseAlignAxisB=+X  BlockFunction=simmechanics.library.frames_transforms.rigid_transform
  Rigidite en torsion : sm_lib/Joints/Revolute Joint  SenseConstraintForceX=off  SenseConstraintForceY=off  SenseConstraintForceZ=off  SenseConstraintTorqueX=off  SenseConstraintTorqueY=off  SenseConstraintTorqueZ=off  ConstraintWrenchDir=FollowerOnBase  ConstraintWrenchFrame=BaseFrame  EquilibriumPosition=0  EquilibriumPositionUnits=rad  SpringStiffness=SimParam.Motor.k  SpringStiffnessUnits=N*m/rad  DampingCoefficient=SimParam.Motor.c2  DampingCoefficientUnits=N*m/(rad/s)  ActuationMode=NoActuation  SensePosition=off  SenseVelocity=off  SenseAcceleration=off  SenseTorqueForce=off  PositionTargetValue=0  PositionTargetValueUnits=rad  PositionTargetSpecify=on  PositionTargetPriority=High  VelocityTargetValue=0  VelocityTargetValueUnits=rad/s  VelocityTargetSpecify=on  VelocityTargetPriority=High  BlockFunction=simmechanics.library.joints.revolute_joint
  Simulink-PS Converter : nesl_utility/Simulink-PS Converter  PhysicalDomain=network_engine_domain  SubClassName=ps_input  LeftPortType=input  RightPortType=output  PseudoPeriodic=off  Frequencies=[]  NoiseDistribution=none  NoiseParameters=[]  Unit=1  AffineConversion=off  InputFiltering=off  SimscapeFilterOrder=1  InputFilterTimeConstant=0.001  UdotUserProvided=1
  Frame : PMIOPort  Port=1  Side=Left
  Arm : PMIOPort  Port=2  Side=Right
  Alpha : Outport
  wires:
  PS-Simulink Converter/1 -> Alpha/1
  Torque/1 -> Simulink-PS Converter/1
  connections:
  Rigidite en torsion/LConn1 -- Motor Inertia 1/RConn1 -- Revolute Joint/RConn1
  Gear/LConn1 -- Motor Inertia 2/2/RConn1 -- Rigidite en torsion/RConn1
  Simulink-PS Converter/RConn1 -- Revolute Joint/LConn2
  PS-Simulink Converter/LConn1 -- Revolute Joint/RConn2
  Revolute Joint2/LConn1 -- Rigid Transform4/LConn1 -- Rigid Transform1/RConn1 -- Revolute Joint/LConn1
  Frame/RConn1 -- Rigid Transform1/LConn1
  Gear1/LConn1 -- Revolute Joint1/RConn1 -- Gear/RConn1 -- Motor Inertia 2/2 _bis/RConn1
  Rigid Transform2/LConn1 -- Revolute Joint2/RConn1 -- Gear1/RConn1
  Revolute Joint1/LConn1 -- Rigid Transform4/RConn1
  Arm/RConn1 -- Rigid Transform2/RConn1
